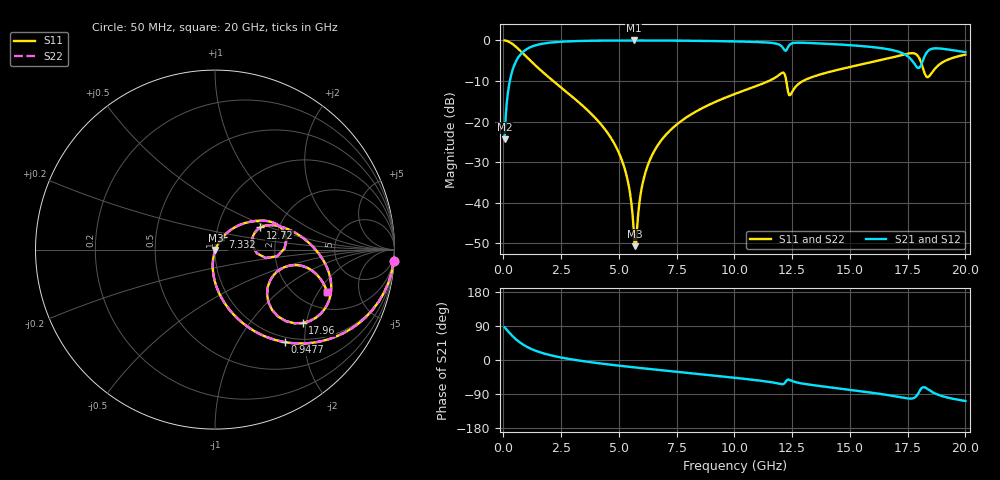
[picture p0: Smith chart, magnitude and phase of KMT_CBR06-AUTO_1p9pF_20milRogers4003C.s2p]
! Data measured by Modelithics Inc. support@modelithics.com 813-866-6335
! KEMET CBR06-AUTO 1.9pF, Pad Width= 0.851mm, Pad Length= 0.64mm, Pad Gap= 0.62mm, 20mil Rogers 4003C substrate Data, January 2022
# hz S ma R 50
! 2 Port Network Data from SP1.SP block
! freq  magS11  angS11  magS21  angS21  magS12  angS12  magS22  angS22
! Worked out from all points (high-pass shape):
!   401 points, 50 MHz to 20 GHz, reference 50 ohm
!   highest |S21| = -0.02 dB at 5.636 GHz (marker M1); lowest = -24.4 dB at 50 MHz (marker M2)
!   |S21| within 3 dB of the highest: 811.9 MHz to 17.22 GHz (16.41 GHz wide, 182 % of centre); 18.32 GHz to end of sweep
!   lowest |S11| = -50.7 dB at 5.686 GHz (marker M3), VSWR 1.01, Z = 50.2 - j0.215 ohm
!   |S11| at or under -10 dB: 2.152 GHz to 11.49 GHz (9.335 GHz wide, 137 % of centre); 12.24 GHz to 12.97 GHz (723.7 MHz wide, 5.74 % of centre)
!   |S22| runs from -50.7 to 0.0 dB; largest |S21 - S12| = 0
!   S11 on the Smith chart (normalised r, x): 50 MHz: 1, -32; 947.8 MHz: 0.91, -1.62; 7.332 GHz: 1.08, +0.15; 12.72 GHz: 1.61, +0.43; 17.96 GHz: 1.38, -1.91; 20 GHz: 2.82, -2.41
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5e7  0.9982 -3.6  0.0603 86.4  0.0603 86.4  0.9982 -3.6
3.4925e8  0.9205 -24.2  0.3898 65.8  0.3898 65.8  0.9205 -24.2
9.4775e8  0.6475 -52.8  0.7607 37.1  0.7607 37.1  0.6475 -52.8
1.8455e9  0.3749 -74.1  0.9252 15.6  0.9252 15.6  0.3749 -74.1
3.391625e9  0.1603 -91.8  0.9848 -2.5  0.9848 -2.5  0.1603 -91.8
5.0375e9  0.03886 -101.6  0.9966 -15.2  0.9966 -15.2  0.03886 -101.6
5.386625e9  0.01837 -99.7  0.9971 -17.6  0.9971 -17.6  0.01837 -99.7
5.636e9  0.004853 -77.1  0.9972 -19.3  0.9972 -19.3  0.004853 -77.1
5.685875e9  0.002921 -47.0  0.9972 -19.6  0.9972 -19.6  0.002921 -47.0
6.13475e9  0.02301 60.8  0.9968 -22.5  0.9968 -22.5  0.02301 60.8
6.73325e9  0.05379 60.7  0.9955 -26.3  0.9955 -26.3  0.05379 60.7
7.33175e9  0.08363 57.9  0.9933 -30.1  0.9933 -30.1  0.08363 57.9
1.0025e10  0.2194 42.0  0.9713 -47.0  0.9713 -47.0  0.2194 42.0
1.206988e10  0.3995 13.0  0.8306 -64.0  0.8306 -64.0  0.3995 13.0
1.2419e10  0.2125 13.5  0.8971 -53.5  0.8971 -53.5  0.2125 13.5
1.271825e10  0.2817 25.9  0.937 -59.5  0.937 -59.5  0.2817 25.9
1.336662e10  0.3538 22.5  0.9257 -66.0  0.9257 -66.0  0.3538 22.5
1.670825e10  0.604 -5.4  0.7733 -93.2  0.7733 -93.2  0.604 -5.4
1.795512e10  0.6368 -40.0  0.4563 -88.5  0.4563 -88.5  0.6368 -40.0
1.825438e10  0.3814 -40.5  0.6554 -72.6  0.6554 -72.6  0.3814 -40.5
1.86035e10  0.421 -12.4  0.7944 -85.8  0.7944 -85.8  0.421 -12.4
2e10  0.6684 -20.7  0.7155 -108.3  0.7155 -108.3  0.6684 -20.7
